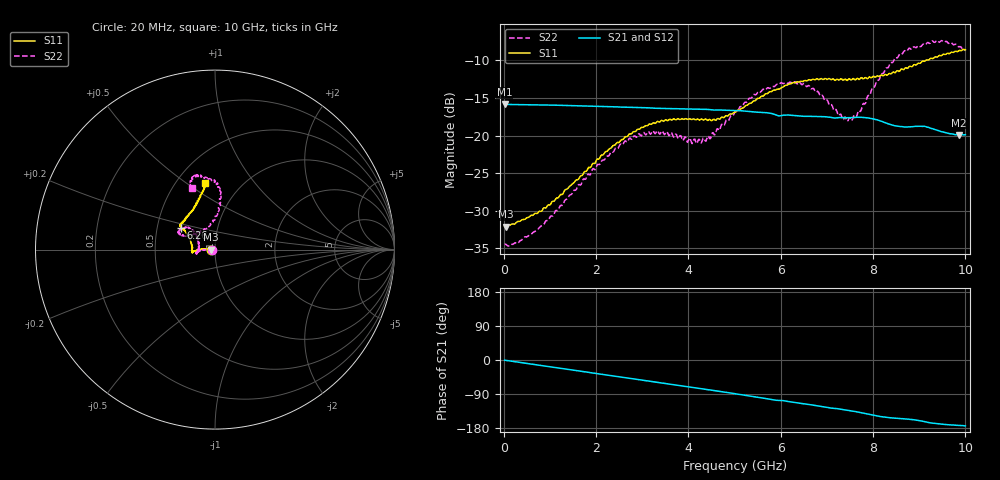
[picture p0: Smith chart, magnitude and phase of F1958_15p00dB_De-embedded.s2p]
! Integrated Device Technology
! Corporate Headquarters
! 6024 Silver Creek Valley Road
! San Jose, CA 95138  USA
! Phone:  1-408-284-8200
! Toll Free:  1-800-223-1366
! Webpage:  http://www.idt.com/
! Timing and RF Division
! 515 Groton Road, Suite 102
! Westford, MA 01886-6024
! Device:  F1958
! Description: 7-bit 0.25 dB Digital Step Attenuator
! Frequency:  0.001 -  6.000 GHz
! Package:  4x4 mm Thin QFN Plastic Package: 24 pin
! Ports:  2 RF, 12 DC
!  Pin  1  = D0
!  Pin  2  = VDD
!  Pin  3  = VMODE
!  Pin  4  = GND
!  Pin  5  = RF1  =  Port 1
!  Pin  6  = GND
!  Pin  7  = GND
!  Pin  8  = GND
!  Pin  9  = GND
!  Pin 10  = GND
!  Pin 11  = GND
!  Pin 12  = GND
!  Pin 13  = GND
!  Pin 14  = RF2  =  Port 2
!  Pin 15  = GND
!  Pin 16  = LE
!  Pin 17  = CLK
!  Pin 18  = DATA
!  Pin 19  = D6
!  Pin 20  = D5
!  Pin 21  = D4
!  Pin 22  = D3
!  Pin 23  = D2
!  Pin 24  = D1
! State:  60
! Atten State:  15.00 dB
! Voltage:  +3.30 Volts
! Current:  0.258 mA
! Data:  The device was measured on a F1958 evaluation board which has
!  individual transmission lines to the RF pins.  Data was collected
!  using a calibrated network analyzer.  The evaluation board was
!  de-embedded using Automatic Fixture Removal (AFR).
!  The reference plane is the edge of the package pin.
! Misc:
!  Action Tracker AT0419
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# GHz S dB R 50
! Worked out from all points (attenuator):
!   500 points, 20 MHz to 10 GHz, reference 50 ohm
!   highest |S21| = -15.83 dB at 20 MHz (marker M1); lowest = -19.9 dB at 9.86 GHz (marker M2)
!   lowest |S11| = -32.1 dB at 40 MHz (marker M3), VSWR 1.05, Z = 47.6 - j0.0729 ohm
!   |S11| at or under -10 dB: start of sweep to 9.14 GHz
!   |S22| runs from -34.7 to -7.3 dB; largest |S21 - S12| = 0.00054
!   S11 on the Smith chart (normalised r, x): 20 MHz: 0.95, -0.00; 6.26 GHz: 0.67, +0.17; 10 GHz: 0.69, +0.59
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0.02  -32.11 -178.1  -15.83 -0.5  -15.83 -0.5  -34.52 -177.9
0.04  -32.13 -178.2  -15.84 -0.8  -15.84 -0.8  -34.46 -176.7
0.3  -31.44 177.2  -15.88 -5.6  -15.88 -5.5  -34.38 179.3
0.72  -30.38 177.0  -15.92 -13.0  -15.91 -13.0  -32.56 179.4
1.7  -25.32 177.1  -16.05 -30.4  -16.04 -30.3  -26.13 179.6
2.6  -20.43 -178.8  -16.21 -46.3  -16.20 -46.3  -20.99 -175.4
2.92  -19.15 -175.9  -16.27 -52.0  -16.25 -52.0  -19.79 -171.9
3.36  -18.19 -173.3  -16.37 -59.7  -16.37 -59.9  -19.65 -167.3
4.3  -17.83 -179.0  -16.50 -76.3  -16.51 -76.3  -20.69 164.4
4.64  -17.71 172.5  -16.60 -82.2  -16.61 -82.2  -19.10 151.7
5.02  -16.90 161.2  -16.65 -89.2  -16.66 -89.2  -16.72 140.5
5.54  -15.01 150.9  -16.90 -98.8  -16.90 -98.8  -14.16 141.7
6.26  -12.97 147.0  -17.32 -111.5  -17.33 -111.5  -13.05 152.8
6.68  -12.54 145.1  -17.45 -118.7  -17.47 -118.6  -13.75 155.5
7.32  -12.46 139.4  -17.62 -130.4  -17.62 -130.3  -17.45 135.4
7.5  -12.49 136.3  -17.62 -133.6  -17.62 -133.5  -17.63 117.5
7.7  -12.54 132.3  -17.57 -138.0  -17.57 -137.9  -16.67 100.5
8.34  -11.75 117.5  -18.46 -152.2  -18.46 -152.3  -10.83 83.5
8.68  -11.10 110.8  -18.86 -155.2  -18.86 -155.3  -8.69 87.9
9.26  -9.70 103.0  -19.05 -166.1  -19.04 -166.1  -7.53 100.6
9.86  -8.70 98.6  -19.92 -172.5  -19.94 -172.5  -8.18 109.8
10  -8.57 98.6  -19.88 -174.0  -19.91 -173.9  -8.67 110.7
